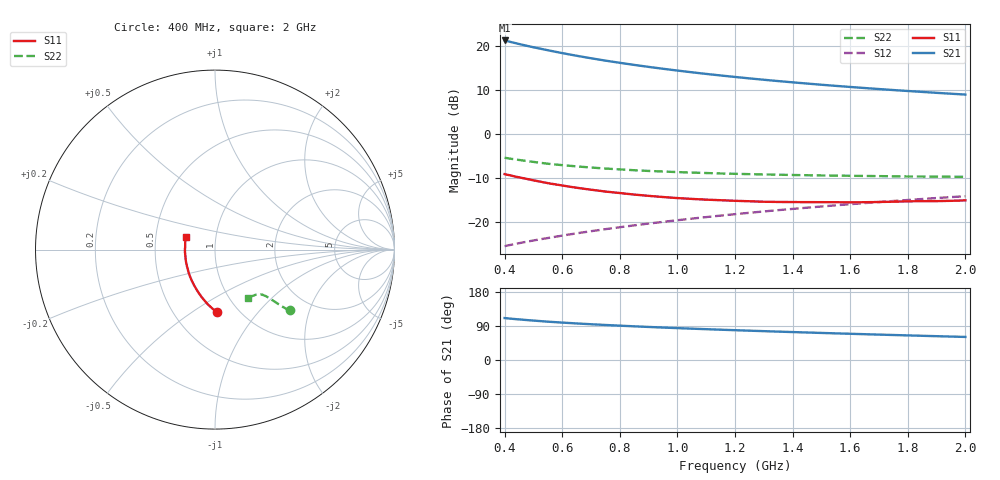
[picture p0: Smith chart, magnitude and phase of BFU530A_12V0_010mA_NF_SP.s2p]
! Filename:  P:\Prog\Test\Noise\ATS_data\Testdata_Net\06 Compressed Noise after Statistics\BFU530A_APG2013_33_A05_12p0V_010mA_NF_CM01_D.sf
! Date/Time: Tue 16/Apr/2013 15:11:03
! BFU530A_APG2013_33_A05_12p0V_1to25mA_NF_CM01_Bias5_R.sf
! Noise Parameter Data File
! BFU530A_APG2013_33_A05_12p0V_1to25mA_NF_CM01
! Date/time: Fri Apr 12 17:55:00 2013
! VAR V_out= 12.001000
! VAR I_out= 9.995000
! VAR V_in= 0.804800
! VAR I_in= 0.090605
! Device data file deembeded for feedlines and parallel
! Original file: \06 Compressed Noise after Statistics\BFU530A_APG2013_33_A05_12p0V_010mA_NF_CM01_R.sf
! Feed-files: PR017V01_150413_Feed1.s2p, PR017V01_150413_Feed2.s2p
! Parallel-file: PR017V01_150413_Par.s2p
# MHz S MA R 50
!  Freq-MHz  S11-mag  S11-arg  S21-mag  S21-arg  S12-mag  S12-arg  S22-mag  S22-arg
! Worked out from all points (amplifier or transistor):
!   37 points, 400 MHz to 2 GHz, reference 50 ohm
!   highest |S21| = 21.3 dB at 400 MHz (marker M1)
!   |S21| within 3 dB of that: start of sweep to 609.8 MHz
!   unconditionally stable (mu >= 1): 1.356 GHz to end of sweep
!   at 500 MHz: K = 0.79, MSG = 22.0 dB, |S12| = -24.2 dB
!   at 1.1 GHz: K = 0.98, MSG = 16.3 dB, |S12| = -18.9 dB
!   at 2 GHz: K = 1.01, MAG = 11.0 dB, |S12| = -14.2 dB
!   lowest NFmin = 0.82 dB at 420 MHz
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400  0.3497 -88.0  11.64 110.7  0.05285 64.6  0.5373 -39.1
420  0.338 -90.6  11.21 109.2  0.0546 64.6  0.5242 -39.5
440  0.3262 -93.1  10.81 107.8  0.05629 64.7  0.5125 -39.8
460  0.3164 -95.3  10.43 106.5  0.05801 64.8  0.5018 -40.0
480  0.3069 -97.6  10.07 105.2  0.05965 64.9  0.491 -40.2
500  0.2973 -99.8  9.738 104.0  0.06137 65.0  0.4818 -40.5
550  0.2759 -105.4  9.009 101.2  0.06544 65.3  0.4592 -40.8
600  0.2593 -110.2  8.356 98.7  0.06973 65.6  0.4425 -41.1
650  0.2446 -115.0  7.794 96.5  0.07401 65.9  0.4282 -41.4
700  0.2323 -119.6  7.301 94.4  0.07825 66.2  0.4158 -41.6
750  0.2214 -124.1  6.862 92.4  0.08253 66.5  0.4047 -41.8
800  0.2129 -128.4  6.478 90.6  0.08686 66.7  0.396 -42.0
850  0.2046 -132.8  6.132 88.9  0.09119 66.9  0.3872 -42.4
950  0.1918 -140.9  5.541 85.7  0.09993 67.1  0.3743 -43.0
1050  0.1825 -148.6  5.053 82.7  0.1088 67.3  0.3639 -43.6
1150  0.1764 -156.0  4.647 80.0  0.1178 67.3  0.3555 -44.5
1200  0.1736 -159.4  4.471 78.7  0.1223 67.3  0.3525 -45.0
1350  0.1685 -169.3  4.012 74.9  0.1359 67.0  0.3445 -46.6
1500  0.1677 -178.7  3.644 71.4  0.1496 66.7  0.3375 -48.5
1650  0.1674 173.2  3.344 68.1  0.1636 66.1  0.3332 -50.6
1750  0.1697 168.0  3.171 66.0  0.1727 65.6  0.3303 -52.0
2000  0.1757 156.9  2.816 60.9  0.196 64.3  0.3259 -56.1
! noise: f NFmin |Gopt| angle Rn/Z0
400  0.8476  0.02987  151.6  0.1015
460  0.8351  0.05037  -178.3  0.092
600  0.8913  0.01334  167  0.1174
800  0.8823  0.07088  175.8  0.0919
1000  0.8889  0.08722  179.2  0.0913
1200  0.9351  0.09175  174.4  0.0933
1400  0.9756  0.1163  -169.2  0.0901
1600  0.9892  0.1441  -159.3  0.089
1800  0.9566  0.1897  -162.9  0.0783
2000  0.9852  0.1928  -153.9  0.0863
